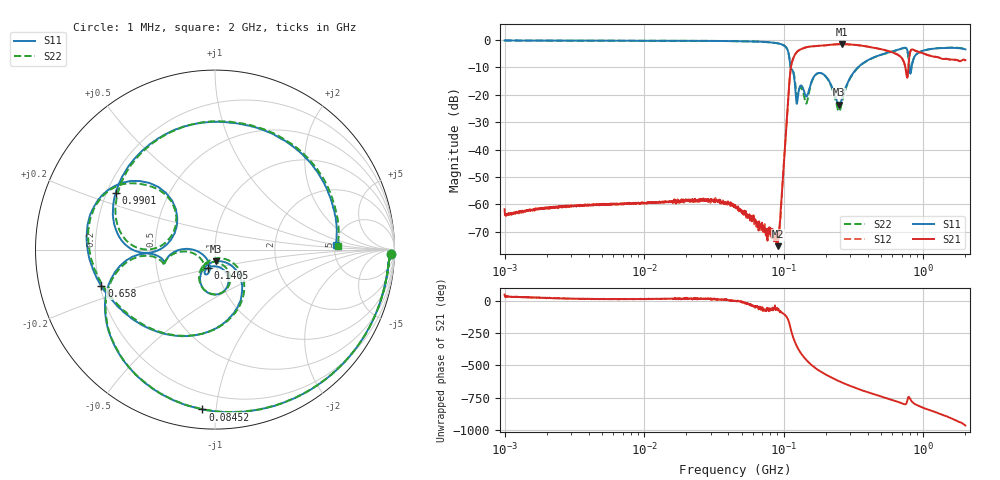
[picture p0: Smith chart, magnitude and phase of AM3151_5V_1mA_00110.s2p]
! Date/Time: Fri Jun 26 10:30:02 2020
! Network Analyzer:  Rev:
! Sweep from 1000000.0 to 2000000000.0, 1601 Points ! Power Supply: 0 V, 0 A
# HZ S DB R 50
!freq MagS11 AngS11 MagS21 AngS21 MagS12 AngS12 MagS22 AngS22
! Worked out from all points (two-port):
!   1601 points, 1 MHz to 2 GHz, reference 50 ohm
!   highest |S21| = -1.51 dB at 259.3 MHz (marker M1); lowest = -75.3 dB at 90.34 MHz (marker M2)
!   |S21| within 3 dB of the highest: 123.5 MHz to 597 MHz (473.6 MHz wide, 131 % of centre); 803.2 MHz to 946.3 MHz (143 MHz wide, 16.4 % of centre)
!   lowest |S11| = -23.6 dB at 248.5 MHz (marker M3), VSWR 1.14, Z = 50.2 - j6.62 ohm
!   |S11| at or under -10 dB: 112 MHz to 340 MHz (228 MHz wide, 101 % of centre); 795.6 MHz to 822.7 MHz (27.12 MHz wide, 3.35 % of centre)
!   |S22| runs from -26.1 to -0.2 dB; largest |S21 - S12| = 0.0097
!   S11 on the Smith chart (normalised r, x): 1 MHz: 37, -47; 84.52 MHz: 0.10, -0.92; 140.5 MHz: 0.90, -0.19; 658 MHz: 0.21, -0.15; 990.1 MHz: 0.24, +0.25; 2 GHz: 5.09, +0.49
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1000000  -0.18 -1.5  -61.79 53.1  -63.73 36.3  -0.18 -1.5
3555161  -0.25 -3.7  -60.27 20.7  -60.43 20.0  -0.25 -3.7
1.263916e7  -0.29 -12.1  -59.35 18.7  -59.25 19.7  -0.29 -12.0
4.493426e7  -0.42 -43.7  -61.24 4.7  -60.93 2.5  -0.41 -43.6
8.452319e7  -0.98 -94.5  -71.86 -54.6  -71.10 -42.5  -0.99 -94.4
9.03357e7  -1.20 -105.5  -75.29 -58.0  -72.55 -57.7  -1.21 -105.3
1.041727e8  -2.75 -146.1  -32.02 -116.8  -32.04 -117.0  -2.76 -145.7
1.129347e8  -10.66 -168.3  -9.41 131.5  -9.42 131.4  -10.50 -165.4
1.259737e8  -21.04 -110.7  -4.05 -4.2  -4.07 -4.1  -20.06 -130.0
1.405178e8  -19.13 -111.8  -2.86 -79.8  -2.86 -80.0  -21.11 -120.4
1.589914e8  -14.88 -65.5  -2.33 -138.7  -2.32 -138.8  -15.07 -61.3
1.904465e8  -12.38 -101.1  -2.03 162.2  -2.04 162.2  -12.45 -101.8
2.4849e8  -23.62 -84.2  -1.54 97.9  -1.56 97.8  -26.13 -84.0
2.593446e8  -21.90 -56.7  -1.51 88.9  -1.51 88.8  -23.49 -47.7
3.721142e8  -8.38 -76.3  -2.15 22.6  -2.18 22.3  -8.48 -74.1
5.652395e8  -4.53 -137.5  -4.10 -40.7  -4.10 -40.7  -4.60 -138.1
6.580422e8  -3.55 -162.3  -5.40 -63.5  -5.41 -63.8  -3.61 -163.9
7.552395e8  -3.01 156.9  -12.16 -76.4  -12.18 -76.2  -3.22 153.7
8.148812e8  -11.43 173.6  -3.67 -51.2  -3.66 -51.1  -11.26 170.8
9.901099e8  -3.92 150.5  -4.82 -108.5  -4.80 -108.2  -3.96 147.4
1.434198e9  -2.93 80.6  -6.88 -171.5  -6.84 -171.4  -2.86 77.3
2e9  -3.42 2.2  -7.39 112.5  -7.54 112.0  -3.29 1.8
